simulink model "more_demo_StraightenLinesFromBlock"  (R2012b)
settings: Solver=ode45  SolverMode=SingleTasking  StartTime=0.0  StopTime=10.0  RelTol=1e-3

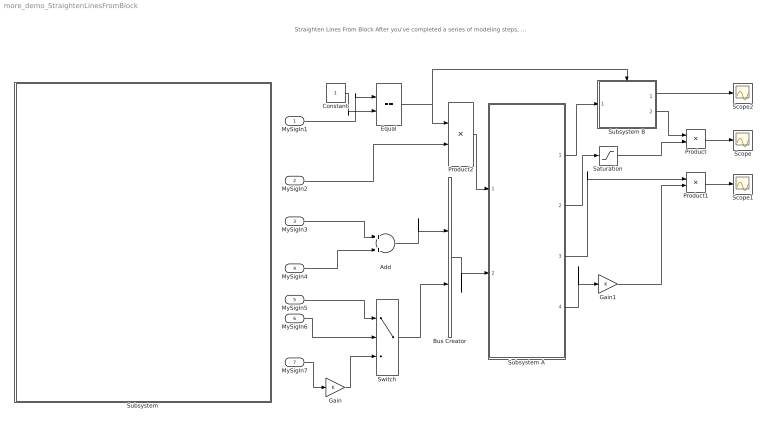
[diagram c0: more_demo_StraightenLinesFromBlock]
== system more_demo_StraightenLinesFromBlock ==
  note: Straighten Lines From Block After you've completed a series of modeling steps, your model may look cluttered. The "Straighten Lines from Block" action helps you to clean up the layout of your model.
  MySigIn1 : Inport
  MySigIn2 : Inport  Port=2
  MySigIn3 : Inport  Port=3
  MySigIn4 : Inport  Port=4
  MySigIn5 : Inport  Port=5
  MySigIn6 : Inport  Port=6
  MySigIn7 : Inport  Port=7
  Add : Sum
  Bus Creator : BusCreator  Inputs=2
  Constant : Constant
  Equal : RelationalOperator  Operator===  OutDataTypeStr=boolean
  Gain : Gain
  Gain1 : Gain
  Product : Product
  Product1 : Product
  Product2 : Product
  Saturation : Saturate
  Scope : Scope
  Scope1 : Scope
  Scope2 : Scope
  Subsystem : Subsystem
  Subsystem A : Subsystem
  Subsystem B : Subsystem  TreatAsAtomicUnit=on
  Switch : Switch  Criteria=u2 > Threshold
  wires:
  MySigIn7/1 -> Gain/1
  Gain/1 -> Switch/3
  MySigIn6/1 -> Switch/2
  MySigIn5/1 -> Switch/1
  Switch/1 -> Bus Creator/2
  MySigIn4/1 -> Add/2
  MySigIn3/1 -> Add/1
  Add/1 -> Bus Creator/1
  Bus Creator/1 -> Subsystem A/2("MySig2 ")
  MySigIn2/1 -> Product2/2
  Constant/1 -> Equal/2
  MySigIn1/1 -> Equal/1
  Equal/1 -> Product2/1, Subsystem B/Enable
  Product2/1 -> Subsystem A/1(MySig1)
  Gain1/1 -> Product1/2
  Subsystem A/4(Result4) -> Gain1/1
  Product1/1 -> Scope1/1
  Subsystem A/3(Result3) -> Product1/1
  Saturation/1 -> Product/2
  Subsystem A/2(Result2) -> Saturation/1
  Product/1 -> Scope/1
  Subsystem B/2(NewResult2) -> Product/1
  Subsystem B/1(NewResult1) -> Scope2/1
  Subsystem A/1(Result1) -> Subsystem B/1(Result1)

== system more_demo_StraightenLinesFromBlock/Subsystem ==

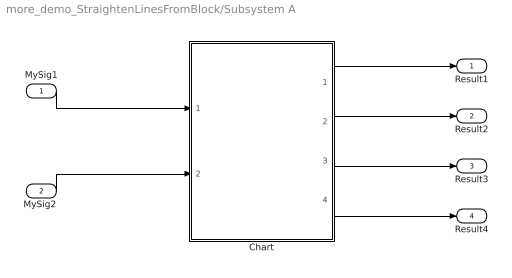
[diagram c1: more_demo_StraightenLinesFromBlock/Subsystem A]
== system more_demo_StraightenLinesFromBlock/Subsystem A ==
  MySig1 : Inport
  "MySig2 " : Inport  Port=2
  Chart : Stateflow chart  TreatAsAtomicUnit=on
  Result1 : Outport
  Result2 : Outport  Port=2
  Result3 : Outport  Port=3
  Result4 : Outport  Port=4
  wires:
  MySig1/1 -> Chart/1(MySig1)
  "MySig2 "/1 -> Chart/2(MySig2)
  Chart/4(Result4) -> Result4/1
  Chart/3(Result3) -> Result3/1
  Chart/2(Result2) -> Result2/1
  Chart/1(Result1) -> Result1/1

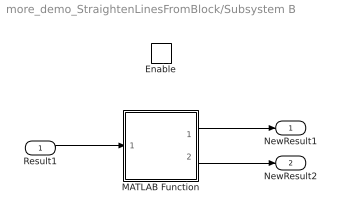
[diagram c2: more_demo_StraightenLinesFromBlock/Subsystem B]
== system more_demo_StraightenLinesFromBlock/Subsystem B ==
  Result1 : Inport
  Enable : EnablePort
  MATLAB Function : MATLAB Function  TreatAsAtomicUnit=on
  NewResult1 : Outport
  NewResult2 : Outport  Port=2
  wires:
  Result1/1 -> MATLAB Function/1(u)
  MATLAB Function/1(y) -> NewResult1/1
  MATLAB Function/2(x) -> NewResult2/1
